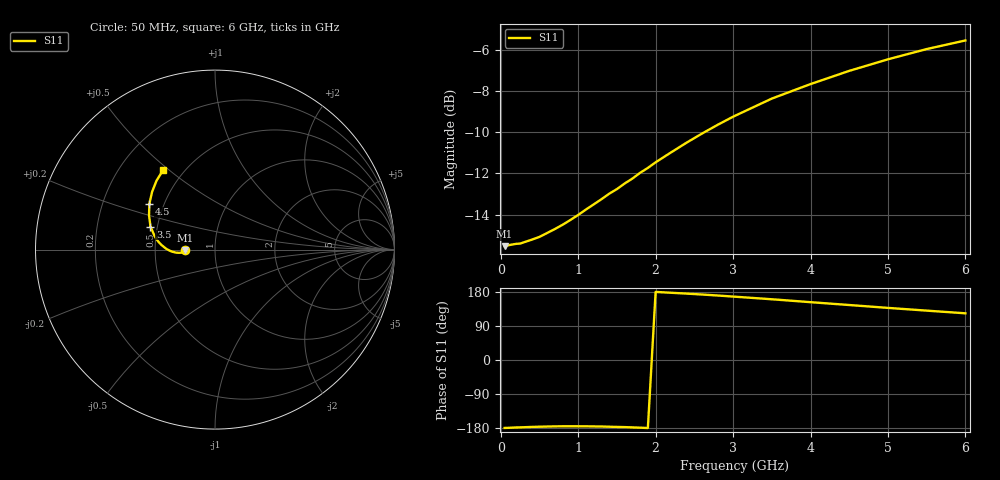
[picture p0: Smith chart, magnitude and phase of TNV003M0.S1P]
! SIEMENS Discrete & RF Semiconductors
! BAS70-07W
! Si Schottky Diode in SOT343
! IF = 3 mA
! S-Parameters:  February  1997
# GHz  S  MA  R  50
!  f  S11
! GHz  MAG  ANG
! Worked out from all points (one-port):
!   34 points, 50 MHz to 6 GHz, reference 50 ohm
!   lowest |S11| = -15.5 dB at 50 MHz (marker M1), VSWR 1.40, Z = 35.7 - j0.15 ohm
!   |S11| at or under -10 dB: start of sweep to 2.629 GHz
!   S11 on the Smith chart (normalised r, x): 50 MHz: 0.71, -0.00; 3.5 GHz: 0.46, +0.14; 4.5 GHz: 0.42, +0.26; 6 GHz: 0.39, +0.48
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0.05  0.1672 -179.3
0.1  0.1681 -179.0
0.2  0.1694 -178.0
0.25  0.1696 -177.7
0.4  0.1734 -176.6
0.5  0.1761 -176.1
0.7  0.184 -175.2
0.8  0.1885 -174.9
1  0.1991 -174.9
1.1  0.2052 -175.0
1.3  0.2174 -175.5
1.4  0.2242 -176.1
1.5  0.2301 -176.6
1.6  0.2374 -177.1
1.7  0.244 -177.8
1.8  0.252 -178.6
1.9  0.2591 -179.5
2  0.2673 179.7
2.4  0.2984 175.2
2.6  0.314 172.8
2.8  0.3296 170.2
3  0.345 167.4
3.5  0.3818 160.3
4  0.414 152.6
4.5  0.4458 145.1
5  0.4756 137.5
5.5  0.5037 130.3
6  0.5285 123.2
